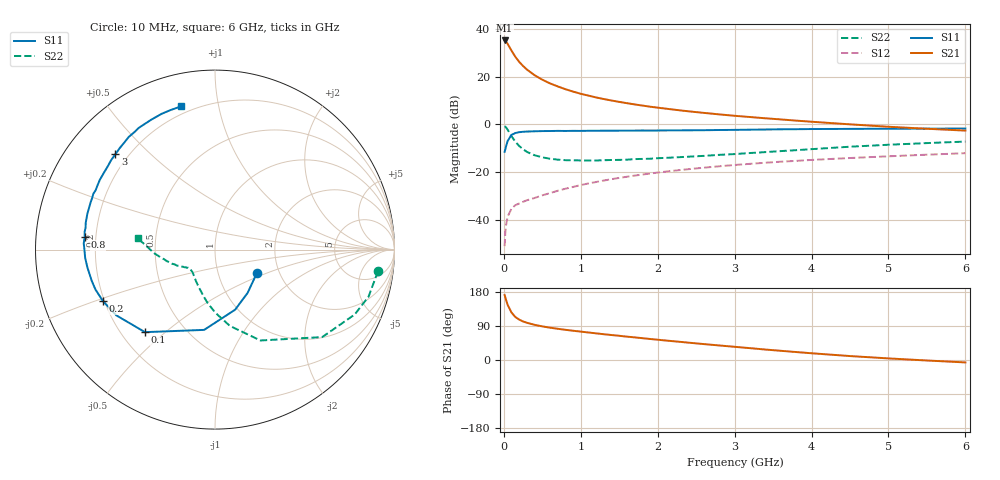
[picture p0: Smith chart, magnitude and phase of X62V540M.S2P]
! SIEMENS Small Signal Semiconductors
! BFP193W
! Si NPN RF Bipolar Junction Transistor in SOT343
! VCE = 2.5 V  IC = 40 mA
! Common Emitter S-Parameters:  April 1994
# GHz  S  MA  R  50
!  f  S11  S21  S12  S22
! GHz  MAG  ANG  MAG  ANG  MAG  ANG  MAG  ANG
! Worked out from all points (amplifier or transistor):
!   40 points, 10 MHz to 6 GHz, reference 50 ohm
!   highest |S21| = 35.2 dB at 10 MHz (marker M1)
!   |S21| within 3 dB of that: start of sweep to 76.97 MHz
!   unconditionally stable (mu >= 1): 647.7 MHz to 3.93 GHz
!   at 200 MHz: K = 0.54, MSG = 29.7 dB, |S12| = -33.2 dB
!   at 1.5 GHz: K = 1.13, MAG = 13.7 dB, |S12| = -22.4 dB
!   at 6 GHz: K = 0.94, MSG = 4.7 dB, |S12| = -12.1 dB
!   S11 on the Smith chart (normalised r, x): 10 MHz: 1.54, -0.42; 100 MHz: 0.30, -0.43; 200 MHz: 0.19, -0.21; 800 MHz: 0.16, +0.05; 3 GHz: 0.15, +0.39; 6 GHz: 0.16, +0.78
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0.01  0.2672 -28.6  57.62 171.5  0.0028 83.7  0.9158 -7.6
0.02  0.3022 -53.1  56.4 164.7  0.0057 76.2  0.8949 -17.0
0.03  0.3531 -71.5  54.45 157.7  0.0079 72.7  0.8584 -24.9
0.05  0.4514 -97.7  48.6 145.3  0.0117 61.1  0.7711 -39.2
0.1  0.603 -130.3  35.13 125.1  0.0172 49.4  0.5662 -63.4
0.15  0.6606 -146.3  26.13 113.4  0.0203 43.9  0.433 -79.0
0.2  0.6871 -155.4  20.46 106.6  0.022 43.6  0.3521 -89.6
0.25  0.7021 -161.5  16.8 101.7  0.0238 44.6  0.3023 -97.6
0.3  0.7086 -165.8  14.12 98.2  0.0257 46.3  0.2654 -104.2
0.4  0.7178 -172.0  10.75 92.8  0.0287 48.6  0.2257 -114.1
0.5  0.7249 -176.4  8.671 88.7  0.0326 52.0  0.2041 -121.5
0.6  0.7273 -179.8  7.25 85.3  0.0363 54.5  0.1909 -127.2
0.8  0.7292 174.5  5.48 79.7  0.0448 58.3  0.1779 -134.4
1.1  0.7357 168.2  4.016 72.6  0.0579 60.4  0.1749 -141.2
1.3  0.7389 164.2  3.403 68.0  0.0666 61.0  0.1776 -143.4
1.6  0.7416 158.9  2.79 61.6  0.08 60.7  0.1825 -146.2
2.2  0.7504 148.7  2.051 49.6  0.1066 58.4  0.2022 -151.9
3  0.7682 136.3  1.517 34.8  0.1411 53.1  0.2389 -159.8
3.2  0.7758 133.1  1.429 31.3  0.1491 51.6  0.2513 -161.7
4.5  0.8062 116.2  1.004 10.4  0.1975 41.9  0.3411 -176.8
5.5  0.8159 107.6  0.811 -1.3  0.2319 35.2  0.4062 174.4
6  0.82 103.3  0.742 -6.4  0.2495 32.3  0.4365 171.2
